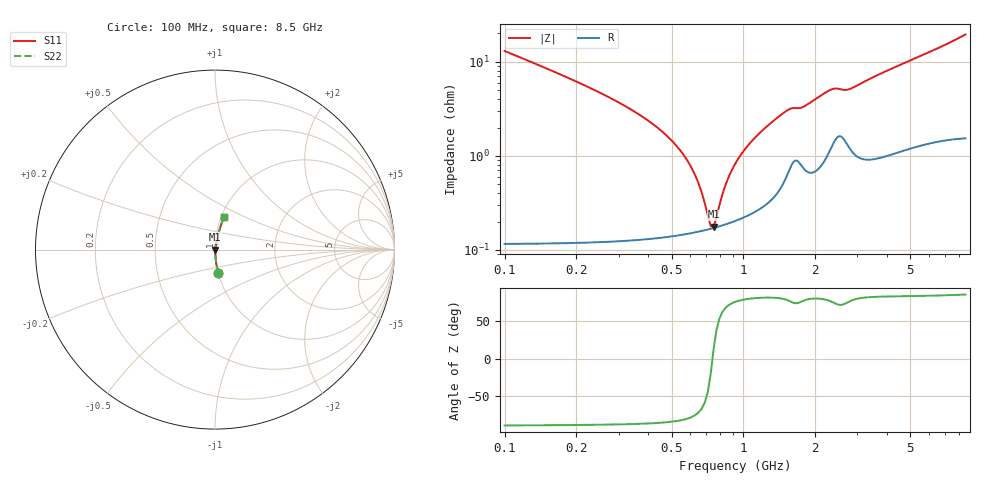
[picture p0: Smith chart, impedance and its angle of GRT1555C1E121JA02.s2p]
!Murata Part Number: GRT1555C1E121JA02
!These Parameters are Measured in Series Mode Connection
!Data Generated on Jun 19, 2026
!  o--ll--o
!Port1  Port2
!  o------o
!Operation Temp=25[degC], DC Bias Voltage=0[V]
!Freq. Start=100[MHz] Stop=9[GHz] 401[Steps]
# Hz S RI R 50
!Freq.(Hz) S11(Real) S11(Imag) S21(Real) S21(Imag) S12(Real) S12(Imag) S22(Real) S22(Imag)
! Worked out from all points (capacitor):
!   401 points, 100 MHz to 8.5 GHz, reference 50 ohm
!   read as one part in series: C = 120 pF near 142 MHz
!   lowest |Z| = 176 mohm at 751 MHz (marker M1)
!   series resonance near 742.4 MHz, so ESL is about 380 pH
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1e8  0.0178 -0.1278  0.9822 0.1278  0.9822 0.1278  0.0178 -0.1278
2.47e8  0.00348 -0.0476  0.9965 0.0476  0.9965 0.0476  0.00348 -0.0476
5.41e8  0.00157 -0.0115  0.9984 0.0115  0.9984 0.0115  0.00157 -0.0115
6.25e8  0.00157 -0.00619  0.9984 0.00619  0.9984 0.00619  0.00157 -0.00619
7.09e8  0.00165 -0.00165  0.9983 0.00165  0.9983 0.00165  0.00165 -0.00165
7.3e8  0.00168 -0.000601  0.9983 0.000601  0.9983 0.000601  0.00168 -0.000601
7.51e8  0.00171 0.000418  0.9983 -0.000418  0.9983 -0.000418  0.00171 0.000418
7.72e8  0.00175 0.00141  0.9983 -0.00141  0.9983 -0.00141  0.00175 0.00141
8.35e8  0.00187 0.00424  0.9981 -0.00424  0.9981 -0.00424  0.00187 0.00424
8.77e8  0.00197 0.00604  0.998 -0.00604  0.998 -0.00604  0.00197 0.00604
9.4e8  0.00214 0.00861  0.9979 -0.00861  0.9979 -0.00861  0.00214 0.00861
1.003e9  0.00233 0.0111  0.9977 -0.0111  0.9977 -0.0111  0.00233 0.0111
1.213e9  0.00324 0.0188  0.9968 -0.0188  0.9968 -0.0188  0.00324 0.0188
1.507e9  0.00666 0.0289  0.9933 -0.0289  0.9933 -0.0289  0.00666 0.0289
1.78e9  0.0084 0.0319  0.9916 -0.0319  0.9916 -0.0319  0.0084 0.0319
2.326e9  0.0142 0.0479  0.9858 -0.0479  0.9858 -0.0479  0.0142 0.0479
2.683e9  0.016 0.0468  0.984 -0.0468  0.984 -0.0468  0.016 0.0468
2.914e9  0.013 0.0518  0.987 -0.0518  0.987 -0.0518  0.013 0.0518
4.3e9  0.0177 0.0844  0.9823 -0.0844  0.9823 -0.0844  0.0177 0.0844
5.707e9  0.0264 0.1144  0.9736 -0.1144  0.9736 -0.1144  0.0264 0.1144
7.114e9  0.0367 0.1464  0.9633 -0.1464  0.9633 -0.1464  0.0367 0.1464
8.5e9  0.05 0.1821  0.95 -0.1821  0.95 -0.1821  0.05 0.1821
